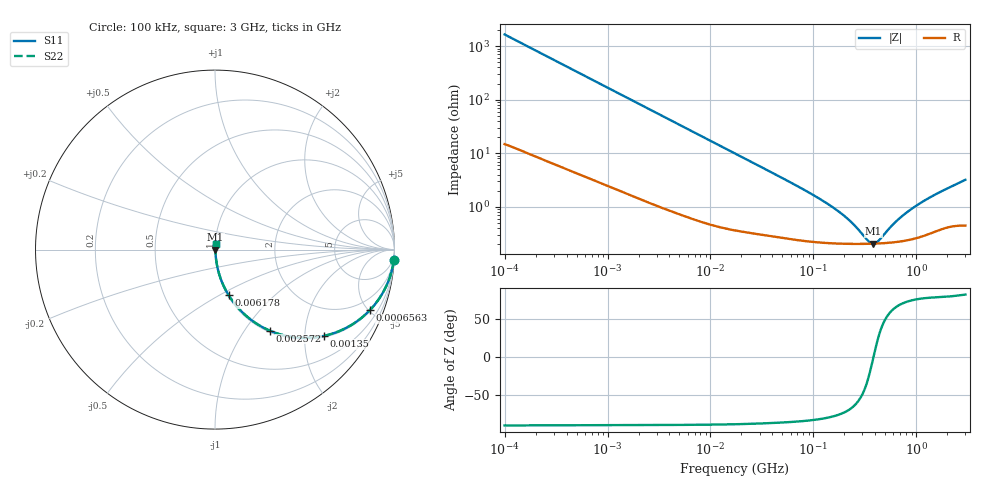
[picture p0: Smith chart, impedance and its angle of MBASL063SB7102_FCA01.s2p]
! MBASL063SB7102_FCA01  S-PARAMETER MODEL  ( Standard Model )
! Model Generated by TAIYO YUDEN Corporation (http://www.ty-top.com)
! Version 1.0
! TAIYO YUDEN Control No. 220601
! Copyright(c) 2020 TAIYO YUDEN CO.,LTD. All Rights Reserved.
! Product Description (link to TY-COMPAS)
! https://ds.yuden.co.jp/TYCOMPAS/or/detail?pn=MBASL063SB7102KFCA01&u=M
! Products Name : Multilayer Ceramic Capacitors
! Characteristics :
!  Capacitance : 1000 [pF] , Rated Voltage : 10 [V] , TCC : X7R
!  Case Size : 0.6 x 0.3 / 0.024 x 0.012 [mm/inch] , Thickness : 0.3 / 0.012 [mm/inch]
!  (Conditions: Temperature = 25 [degC] , DC Bias Voltage = 0 [V])
! External Node Assignments :
!  1  o---| |---o  2
! GND o---------o GND
! Frequency Range : 100kHz  -  3GHz  [ 401 STEP ]
# MHZ S RI R 50
! Freq[MHz].  S11 Real  S11 Imag  S21 Real  S21 Imag  S12 Real  S12 Imag  S22 Real  S22 Imag
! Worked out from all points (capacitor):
!   401 points, 100 kHz to 3 GHz, reference 50 ohm
!   read as one part in series: C = 965 pF near 105.3 kHz
!   lowest |Z| = 206 mohm at 381.7 MHz (marker M1)
!   series resonance near 383.6 MHz, so ESL is about 180 pH
!   S11 on the Smith chart (normalised r, x): 100 kHz: 1, -33; 656.3 kHz: 1.07, -5.08; 1.35 MHz: 1.04, -2.49; 2.572 MHz: 1.02, -1.31; 6.178 MHz: 1.01, -0.55; 3 GHz: 1.01, +0.06
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0.1  0.9958 -0.0605  0.00422 0.0605  0.00422 0.0605  0.9958 -0.0605
0.246461  0.9768 -0.1451  0.0232 0.1451  0.0232 0.1451  0.9768 -0.1451
0.562235  0.8947 -0.3005  0.1053 0.3005  0.1053 0.3005  0.8947 -0.3005
0.656258  0.8627 -0.3375  0.1373 0.3375  0.1373 0.3375  0.8627 -0.3375
0.941399  0.7564 -0.422  0.2436 0.422  0.2436 0.422  0.7564 -0.422
1.350433  0.6056 -0.4809  0.3944 0.4809  0.3944 0.4809  0.6056 -0.4809
1.839868  0.4566 -0.4898  0.5434 0.4898  0.5434 0.4898  0.4566 -0.4898
2.572132  0.3046 -0.4514  0.6954 0.4514  0.6954 0.4514  0.3046 -0.4514
3.161081  0.2271 -0.4097  0.7729 0.4097  0.7729 0.4097  0.2271 -0.4097
6.178009  0.0757 -0.2533  0.9243 0.2533  0.9243 0.2533  0.0757 -0.2533
17.7727  0.0127 -0.095  0.9873 0.095  0.9873 0.095  0.0127 -0.095
97.38194  0.0025 -0.0169  0.9975 0.0169  0.9975 0.0169  0.0025 -0.0169
190.323  0.0021 -0.00699  0.9979 0.00699  0.9979 0.00699  0.0021 -0.00699
246.2744  0.00205 -0.00422  0.998 0.00422  0.998 0.00422  0.00205 -0.00422
344.2911  0.00204 -0.000998  0.998 0.000998  0.998 0.000998  0.00204 -0.000998
381.6779  0.00205 -4.61e-05  0.9979 4.61e-05  0.9979 4.61e-05  0.00205 -4.61e-05
434.1712  0.00208 0.00114  0.9979 -0.00114  0.9979 -0.00114  0.00208 0.00114
547.5153  0.00215 0.00334  0.9979 -0.00334  0.9979 -0.00334  0.00215 0.00334
726.971  0.00232 0.00628  0.9977 -0.00628  0.9977 -0.00628  0.00232 0.00628
1070.062  0.00282 0.0111  0.9972 -0.0111  0.9972 -0.0111  0.00282 0.0111
1658.39  0.00397 0.018  0.996 -0.018  0.996 -0.018  0.00397 0.018
3000  0.00544 0.0314  0.9946 -0.0314  0.9946 -0.0314  0.00544 0.0314
